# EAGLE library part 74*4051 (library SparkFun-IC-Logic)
NXP 74HC4051 8-Channel Analog Multiplexer/Demultiplexer The 74HC4051; 74HCT4051 is a single-pole octal-throw analog switch (SP8T) suitable for use in analog or digital 8:1 multiplexer/demultiplexer applications. The switch features three digital select inputs (S0, S1 and S2), eight independent inputs/outputs (Yn), a common input/output (Z) and a digital enable input (E). When E is HIGH, the switches are turned off. Inputs include clamp diodes. This enables the use of current limiting resistors to interface inputs to voltages in excess of VCC. Datasheet
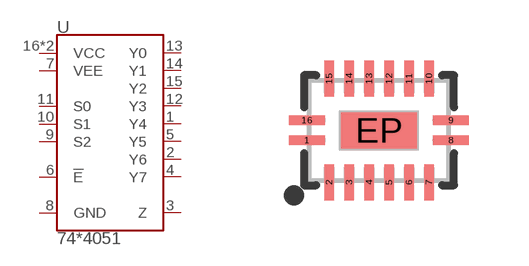
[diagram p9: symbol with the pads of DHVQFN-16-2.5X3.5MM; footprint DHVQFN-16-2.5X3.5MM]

Designator prefix U

## 74HC4051BQ (PROD_ID: IC-13334)  [DHVQFN-16-2.5X3.5MM]
1  Y4
2  Y6
3  Z
4  Y7
5  Y5
6  !E!
7  VEE
8  GND
9  S2
10  S1
11  S0
12  Y3
13  Y0
14  Y1
15  Y2
16  VCC
EP  VCC

## Footprint DHVQFN-16-2.5X3.5MM (pad centres in mm)
16-Pin DHVQFN (SOT763-1) - 2.5 x 3.5 x 0.85 mm Package used by NXP 74HC4051BQ 8-channel analog mux/demux. NXP Footprint for reflow soldering Example Datasheet
smd 0.9 x 0.24: 1 -1.8,-0.25; 8 1.8,-0.25; 9 1.8,0.25; 16 -1.8,0.25
smd 0.24 x 0.9: 2 -1.25,-1.3; 3 -0.75,-1.3; 4 -0.25,-1.3; 5 0.25,-1.3; 6 0.75,-1.3; 7 1.25,-1.3; 10 1.25,1.3; 11 0.75,1.3; 12 0.25,1.3; 13 -0.25,1.3; 14 -0.75,1.3; 15 -1.25,1.3
smd 1.9 x 0.9: EP 0,0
